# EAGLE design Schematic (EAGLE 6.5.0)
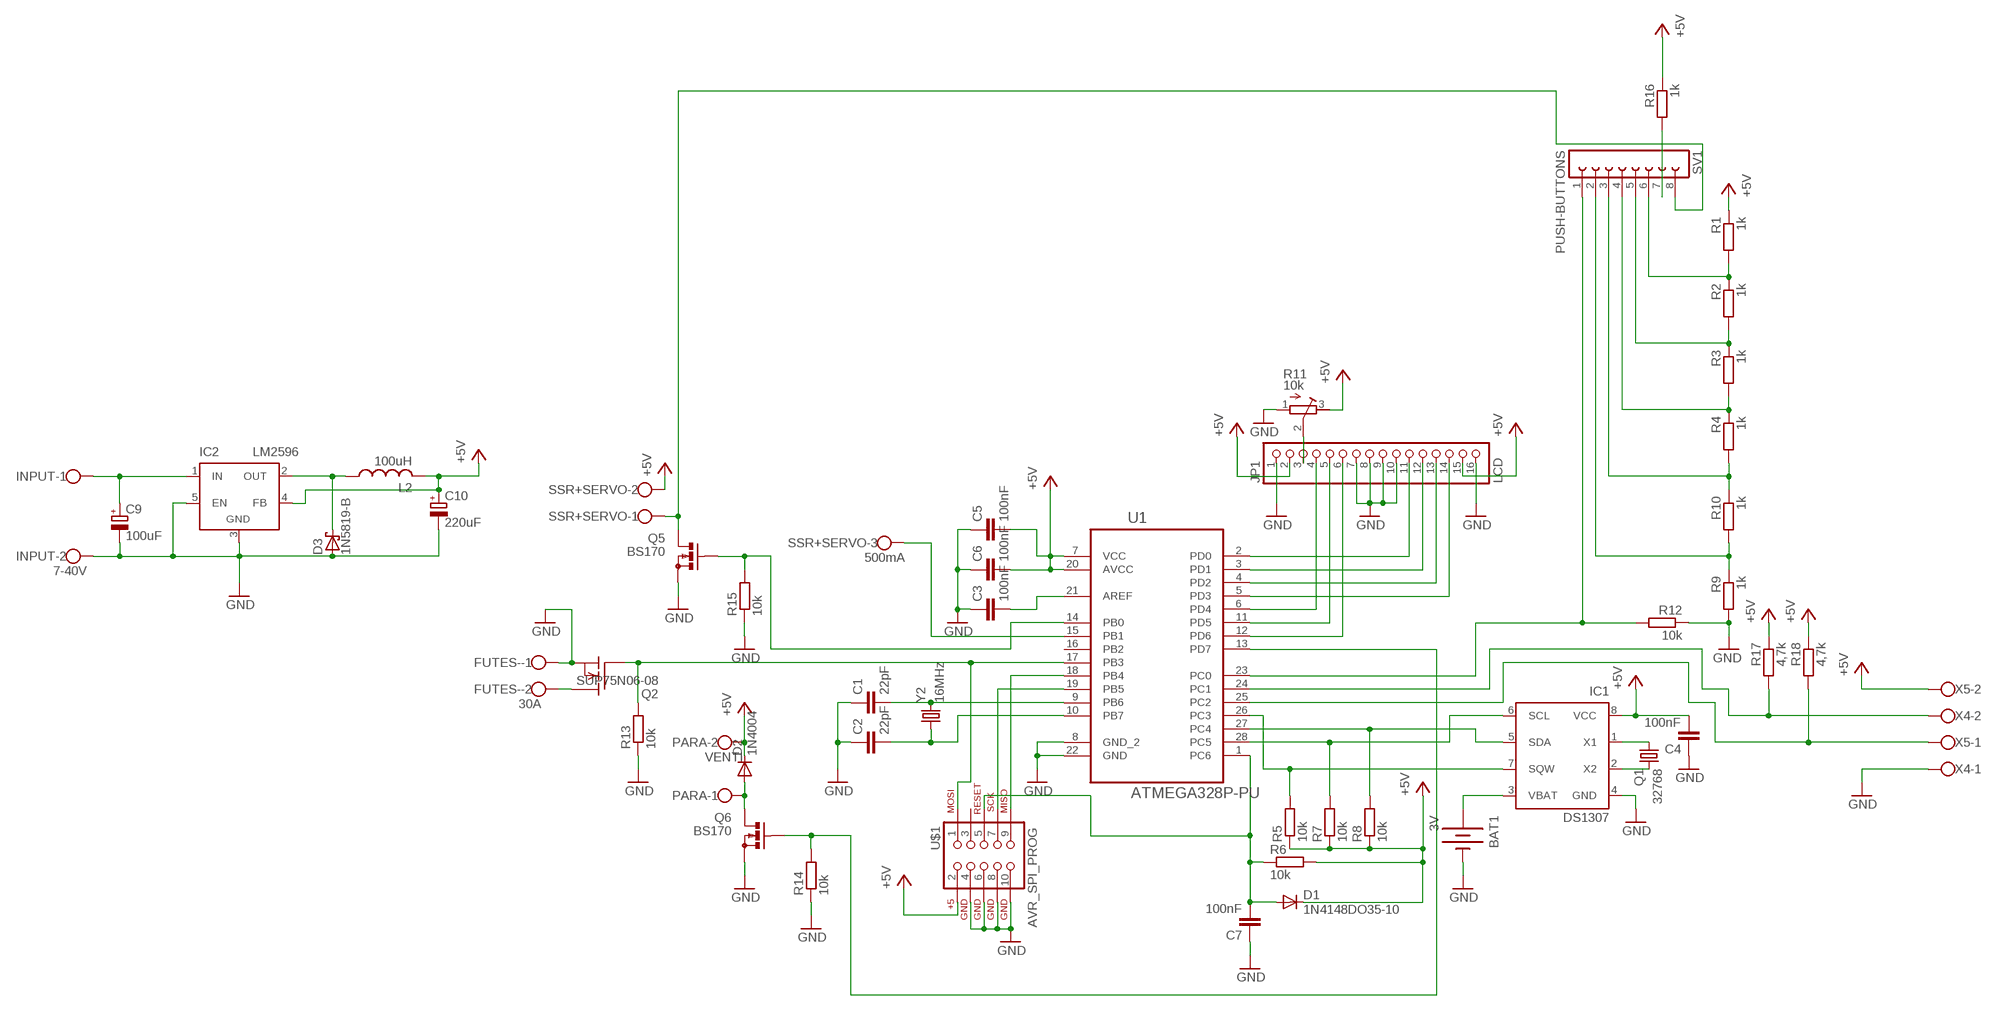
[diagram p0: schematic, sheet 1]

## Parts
BAT1  3V  BATTERY20PTH  [BATTCOM_20MM_PTH]
C1  22pF  CAPKIT  [CAP-PTH-SMALL-KIT]
C2  22pF  CAPKIT  [CAP-PTH-SMALL-KIT]
C3  100nF  CAPKIT  [CAP-PTH-SMALL-KIT]
C4  100nF  CAPKIT  [CAP-PTH-SMALL-KIT]
C5  100nF  CAPKIT  [CAP-PTH-SMALL-KIT]
C6  100nF  CAPKIT  [CAP-PTH-SMALL-KIT]
C7  100nF  CAPKIT  [CAP-PTH-SMALL-KIT]
C9  100uF  CPOL-EUE3.5-8  [E3,5-8]
C10  220uF  CPOL-EUE3.5-8  [E3,5-8]
D1  1N4148DO35-10  [DO35-10]
D2  1N4004  [DO41-10]
D3  1N5819-B  [DO41-7.6]
FUTES-  30A  W237-102  [W237-102]
IC1  DS1307  [DIL08]
IC2  LM2596  LM2596TH  [TO220-52]
INPUT  7-40V  W237-102  [W237-102]
JP1  LCD  PINHD-1X16  [1X16]
L2  100uH  L-US6000-XXX-RC  [6000-XXXX-RC]
PARA  VENTI  W237-102  [W237-102]
Q1  32768  CRYSTALTC26V  [TC26V]
Q2  SUP75N06-08  [TO220]
Q5  BS170  [SOT54E]
Q6  BS170  [SOT54E]
R1  1k  R-EU_0309/10  [0309/10]
R2  1k  R-EU_0309/10  [0309/10]
R3  1k  R-EU_0309/10  [0309/10]
R4  1k  R-EU_0309/10  [0309/10]
R5  10k  R-EU_0309/10  [0309/10]
R6  10k  R-EU_0309/10  [0309/10]
R7  10k  R-EU_0309/10  [0309/10]
R8  10k  R-EU_0309/10  [0309/10]
R9  1k  R-EU_0309/10  [0309/10]
R10  1k  R-EU_0309/10  [0309/10]
R11  10k  R-TRIMM74W  [RTRIM74W]
R12  10k  R-EU_0309/10  [0309/10]
R13  10k  R-EU_0309/10  [0309/10]
R14  10k  R-EU_0309/10  [0309/10]
R15  10k  R-EU_0309/10  [0309/10]
R16  1k  R-EU_0309/10  [0309/10]
R17  4,7k  R-EU_0309/10  [0309/10]
R18  4,7k  R-EU_0309/10  [0309/10]
SSR+SERVO  500mA  W237-103  [W237-103]
SV1  PUSH-BUTTONS  FE08-1  [FE08]
U1  ATMEGA328P-PU  [DIP254P762X457-28]
U$1  AVR_SPI_PROG  [AVR_ICSP]
X4  W237-102  [W237-102]
X5  W237-102  [W237-102]
Y2  16MHz  CRYSTALHC49US  [HC49US]

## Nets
GND: BAT1.2(-) C1.1 C2.1 C3.1 C4.1 C5.1 C6.1 C7.1 C9.- C10.- D3.A FUTES-.1 IC1.4(GND) IC2.3(GND) IC2.5(EN) INPUT.2 JP1.1 JP1.7 JP1.8 JP1.9 JP1.10 JP1.16 Q2.3(S) Q5.S Q6.S R9.2 R11.1(E) R12.1 R13.1 R14.1 R15.1 U1.8(GND_2) U1.22(GND) U$1.4 U$1.6 U$1.8 U$1.10 X4.1
N$1: IC1.6(SCL) R7.2 U1.28(PC5)
N$2: IC1.5(SDA) R8.2 U1.27(PC4)
N$3: IC1.7(SQW) R5.2 U1.26(PC3)
N$4: IC1.2(X2) Q1.2
N$5: IC1.1(X1) Q1.1
N$6: BAT1.1(+) IC1.3(VBAT)
N$7: C1.2 U1.9(PB6) Y2.2
N$8: C2.2 U1.10(PB7) Y2.1
N$9: C3.2 U1.21(AREF)
N$10: JP1.11 U1.2(PD0)
N$11: JP1.12 U1.3(PD1)
N$12: JP1.13 U1.4(PD2)
N$13: JP1.14 U1.5(PD3)
N$14: JP1.4 U1.6(PD4)
N$15: JP1.5 U1.11(PD5)
N$16: JP1.6 U1.12(PD6)
N$17: U1.18(PB4) U$1.9
N$18: C7.2 D1.A R6.1 U1.1(PC6) U$1.5
N$19: U1.19(PB5) U$1.7
N$20: Q2.1(G) R13.2 U1.17(PB3) U$1.1
N$21: C9.+ IC2.1(IN) INPUT.1
N$22: FUTES-.2 Q2.2(D)
N$23: R12.2 SV1.1 U1.23(PC0)
N$24: JP1.3 R11.2(S)
N$25: R3.2 R4.1 SV1.4
N$26: R2.2 R3.1 SV1.5
N$27: R1.2 R2.1 SV1.6
N$28: R9.1 R10.2 SV1.2
N$29: R4.2 R10.1 SV1.3
N$30: Q5.G R15.2 U1.14(PB0)
N$31: Q5.D SSR+SERVO.1 SV1.8
N$32: R16.2 SV1.7
N$33: R17.2 U1.24(PC1) X4.2
N$34: D2.A PARA.1 Q6.D
N$35: R18.2 U1.25(PC2) X5.1
N$36: SSR+SERVO.3 U1.15(PB1)
N$37: D3.C IC2.2(OUT) L2.1
N$38: Q6.G R14.2 U1.13(PD7)
VCC: C4.2 C5.2 C6.2 C10.+ D1.C D2.C IC1.8(VCC) IC2.4(FB) JP1.2 JP1.15 L2.2 PARA.2 R1.1 R5.1 R6.2 R7.1 R8.1 R11.3(A) R16.1 R17.1 R18.1 SSR+SERVO.2 U1.7(VCC) U1.20(AVCC) U$1.2 X5.2 ; supply symbol labelled +5V
Unconnected: U1.16(PB2) U$1.3

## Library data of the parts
BAT1 = SparkFun-Electromechanical:BATTERY: Battery Holders
C1-C7 = SparkFun-Capacitors:CAP: Capacitor
C9 C10 = rcl:CPOL-EU: POLARIZED CAPACITOR, European symbol
D1 = diode:1N4148: DIODE
D2 = diode:1N4004: DIODE
D3 = diode:1N581*: 1.0A SCHOTTKY BARRIER RECTIFIER
FUTES- INPUT PARA X4 X5 = con-wago-500:W237-102: WAGO SCREW CLAMP; MPN: 237-102; OC_FARNELL: unknown; OC_NEWARK: 70K9898
IC1 = ds1307_pcf8583:DS1307: I2C-Bus CLOCK/CALENDAR
IC2 = linear:LM2596T: STEP-DOWN VOLTAGE REGULATOR
JP1 = pinhead:PINHD-1X16: PIN HEADER
L2 = rcl:L-US: INDUCTOR, American symbol
Q1 = crystal:CRYSTAL: CRYSTAL; OC_FARNELL: unknown; OC_NEWARK: unknown
Q2 = transistor-fet:SUP75N06-08: N-Channel Enhancement MOSFET 60V; 75A; 0,008Ohm
Q5 Q6 = transistor-small-signal:BS170: N-CHANNEL MOS FET
R1-R10 R12-R18 = rcl:R-EU_: RESISTOR, European symbol
R11 = resistor:R-TRIMM: Trimm resistor
SSR+SERVO = con-wago-500:W237-103: WAGO SCREW CLAMP; MPN: 237-103; OC_FARNELL: unknown; OC_NEWARK: 18M7116
SV1 = con-lsta:FE08-1: FEMALE HEADER; OC_FARNELL: unknown; OC_NEWARK: unknown
U1 = Atmel_By_element14_Batch_1-00:ATMEGA328P-PU: 8-bit Microcontroller with In-System Programmable Flash; MPN: ATMEGA328P-PU; OC_FARNELL: 1715487; OC_NEWARK: 15R0268; PACKAGE: PDIP-28; SUPPLIER: Atmel
U$1 = SparkFun-Connectors:AVR_SPI_PROG: AVR 10-pin ICSP Header This is the standard AVR In Circuit Serial Programming header. Minimal, but includes pin one indicator. Works with standard Olimex programmers. Also look for the 6-pin reduced version. Spark Fun Electronics SKU: PRT-00778
Y2 = SparkFun-FreqCtrl:CRYSTAL: Various standard crystals. Proven footprints. Spark Fun Electronics SKU : COM-00534

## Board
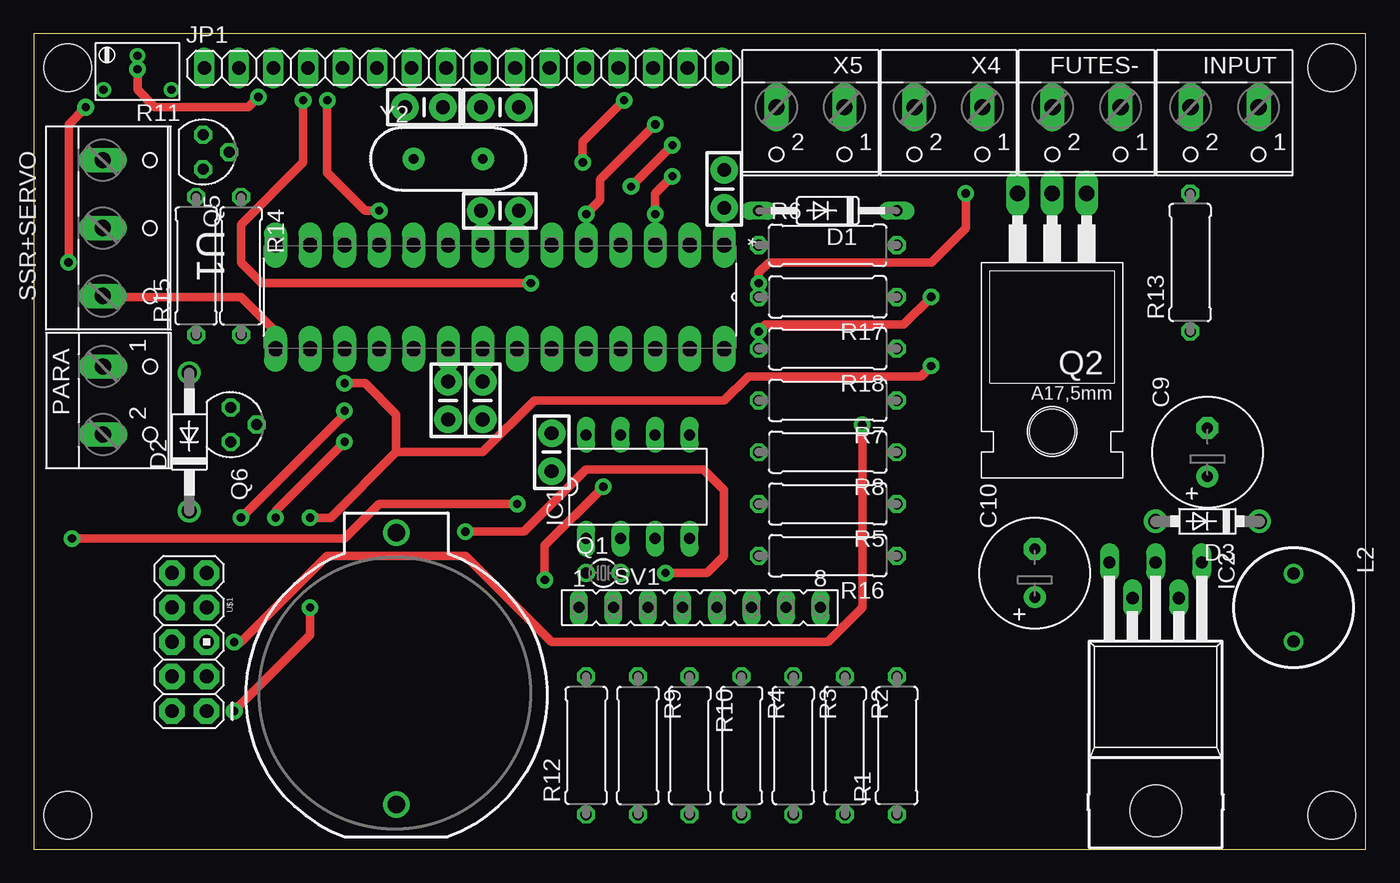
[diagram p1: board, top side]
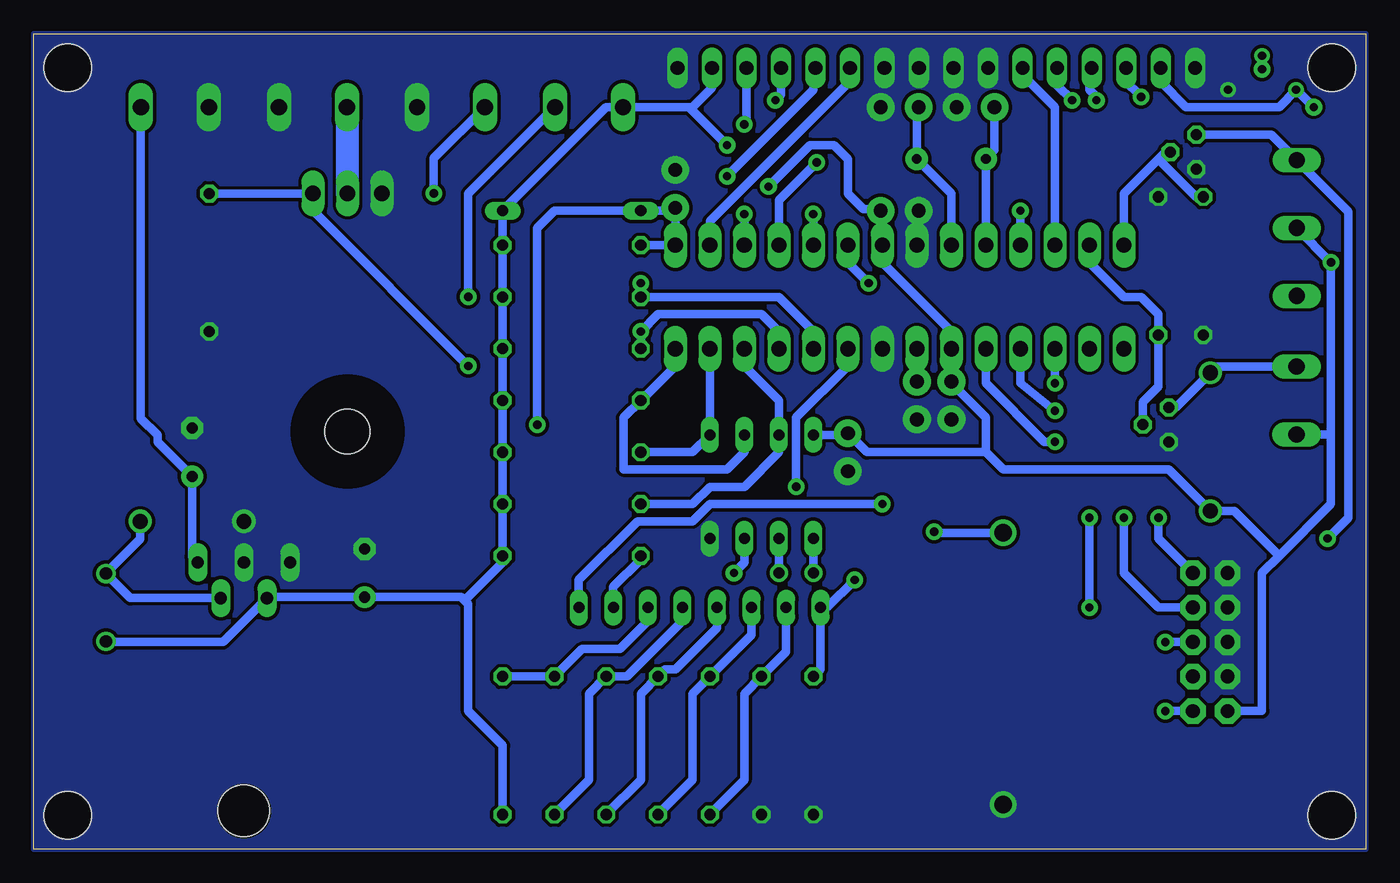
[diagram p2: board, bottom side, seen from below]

Size 98 x 60 mm. Coordinates in mm from the lower left corner, seen from the top.
Outline: 0,0 98,0 98,60 0,60 0,0
Copper layers (1*16): Top 0.035mm / dielectric 1.5mm / Bottom 0.035mm
Design rules "default *": minimum track width 24mil, minimum drill 24mil, track to track 10mil, track to pad 10mil, pad to pad 8mil, via to via 8mil, smd to smd 8mil, copper to edge 0mil, drill to drill 8mil, minimum pad ring 10mil, minimum via ring 12mil, stop-mask expansion 0mil, vias tented up to drill 0mil, thermal gap 10mil
Holes 3.5 mm at 2.5,57.5 95.5,57.5 2.5,2.5 95.5,2.5

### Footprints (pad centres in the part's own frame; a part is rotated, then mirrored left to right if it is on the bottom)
BATTCOM_20MM_PTH = drill 1.3: 1 11.85,0; 2 -8.15,0
CAP-PTH-SMALL-KIT = drill 1.016 pad 2.032: 1 -1.397,0; 2 1.397,0
E3,5-8 = drill 0.813 pad 1.6: + -1.778,0 | drill 0.813 pad 1.6 octagon: - 1.778,0
DO35-10 = drill 0.813 long: A 5.08,0; C -5.08,0
DO41-10 = drill 1.118: A 5.08,0; C -5.08,0
DO41-7.6 = drill 1.1 pad 1.7: A 3.81,0; C -3.81,0
W237-102 = drill 1.194 long: 1 -2.5,-1.27; 2 2.5,-1.27
DIL08 = drill 0.813 long: 1 -3.81,-3.81; 2 -1.27,-3.81; 3 1.27,-3.81; 4 3.81,-3.81; 5 3.81,3.81; 6 1.27,3.81; 7 -1.27,3.81; 8 -3.81,3.81
TO220-52 = drill 0.9 long: 1 -3.4,-21.1; 2 -1.7,-18.47; 3 0,-21.1; 4 1.7,-18.47; 5 3.4,-21.1 | hole 3.8: 0,-2.8
1X16 = drill 1.016 long: 1 -19.05,0; 2 -16.51,0; 3 -13.97,0; 4 -11.43,0; 5 -8.89,0; 6 -6.35,0; 7 -3.81,0; 8 -1.27,0; 9 1.27,0; 10 3.81,0; 11 6.35,0; 12 8.89,0; 13 11.43,0; 14 13.97,0; 15 16.51,0; 16 19.05,0
6000-XXXX-RC = drill 0.9 pad 1.422: 1 -2.5,0; 2 2.5,0
TC26V = drill 0.813: 1 -1.27,0; 2 1.27,0
TO220 = drill 1.118 long: 1 -2.54,-6.35; 2 0,-6.35; 3 2.54,-6.35 | hole 3.302: 0,11.176
SOT54E = drill 0.813 octagon: D -1.27,0; G 0,1.905; S 1.27,0
0309/10 = drill 0.813 octagon: 1 -5.08,0; 2 5.08,0
RTRIM74W = drill 0.61: 1 -1.25,-2.5; 2 1.25,0; 3 -1.25,2.5
W237-103 = drill 1.194 long: 1 -5,-1.29; 2 0,-1.29; 3 5,-1.29
FE08 = drill 0.813 long: 1 -8.89,0; 2 -6.35,0; 3 -3.81,0; 4 -1.27,0; 5 1.27,0; 6 3.81,0; 7 6.35,0; 8 8.89,0
DIP254P762X457-28 = drill 1.118 long: 1 -7.62,33.02; 2 -7.62,30.48; 3 -7.62,27.94; 4 -7.62,25.4; 5 -7.62,22.86; 6 -7.62,20.32; 7 -7.62,17.78; 8 -7.62,15.24; 9 -7.62,12.7; 10 -7.62,10.16; 11 -7.62,7.62; 12 -7.62,5.08; 13 -7.62,2.54; 14 -7.62,0; 15 0,0; 16 0,2.54; 17 0,5.08; 18 0,7.62; 19 0,10.16; 20 0,12.7; 21 0,15.24; 22 0,17.78; 23 0,20.32; 24 0,22.86; 25 0,25.4; 26 0,27.94; 27 0,30.48; 28 0,33.02
AVR_ICSP = drill 1.016 pad 1.88 octagon: 1 -1.27,5.08; 2 1.27,5.08; 3 -1.27,2.54; 4 1.27,2.54; 5 -1.27,0; 6 1.27,0; 7 -1.27,-2.54; 8 1.27,-2.54; 9 -1.27,-5.08; 10 1.27,-5.08
HC49US = drill 0.7 pad 1.651: 1 -2.54,0; 2 2.54,0

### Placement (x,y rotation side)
BAT1  26.67,11.43 90 top
C1  34.29,54.61 180 top
C2  28.7,54.61 180 top
C3  33.02,33.02 90 top
C4  38.1,29.21 90 top
C5  34.29,46.99 0 top
C6  30.48,33.02 90 top
C7  50.8,48.59 270 top
C9  86.36,29.21 90 top
C10  73.66,20.32 90 top
D1  58.42,46.99 180 top
D2  11.43,29.97 90 top
D3  86.36,24.13 180 top
FUTES-  77.47,53.34 180 top
IC1  44.45,26.67 0 top
IC2  82.55,0 180 top
INPUT  87.63,53.34 180 top
JP1  31.59,57.5 0 top
L2  92.71,17.78 270 top
PARA  6.35,33.02 270 top
Q1  41.91,20.32 0 top
Q2  74.93,41.91 180 top
Q5  12.45,51.31 270 top
Q6  14.48,31.24 270 top
R1  63.5,7.62 90 top
R2  59.69,7.62 270 top
R3  55.88,7.62 270 top
R4  52.07,7.62 270 top
R5  58.42,25.4 180 top
R6  58.42,44.45 0 top
R7  58.42,33.02 180 top
R8  58.42,29.21 180 top
R9  44.45,7.62 270 top
R10  48.26,7.62 270 top
R11  7.62,57.15 90 top
R12  40.64,7.62 90 top
R13  85.09,43.18 90 top
R14  15.24,42.93 270 top
R15  11.94,42.93 90 top
R16  58.42,21.59 180 top
R17  58.42,40.64 180 top
R18  58.42,36.83 180 top
SSR+SERVO  6.35,45.72 270 top
SV1  49,17.78 0 top
U1  17.78,36.83 270 top
U$1  11.43,15.24 180 top
X4  67.31,53.34 180 top
X5  57.15,53.34 180 top
Y2  30.48,50.8 0 top

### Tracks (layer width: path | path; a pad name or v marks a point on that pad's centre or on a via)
GND
  pour Bottom (no thermals): 0,0 0,60 98,60 98,0
N$1
  Bottom 0.61: IC1.6 45.72,29.21 46.99,27.94 54.61,27.94 54.61,31.75 R7.2 50.8,35.56 U1.28
N$2
  Bottom 0.61: U1.27 IC1.5 49.53,29.21 R8.2
N$3
  Bottom 0.61: U1.26 45.72,35.56 43.18,33.02 IC1.7 43.18,29.21 45.72,26.67 48.26,26.67 49.53,25.4 R5.2
N$4
  Bottom 0.61: IC1.2 Q1.2
N$5
  Bottom 0.61: IC1.1 Q1.1
N$6  (via drill 0.61)
  Top 0.61: v46.48,20.32 49.53,20.32 50.8,21.59 50.8,26.42 49.28,27.94 40.64,27.94 36.07,23.37 v31.75,23.37
  Bottom 0.61: IC1.3 45.72,21.08 v46.48,20.32 | BAT1.1 31.66,23.28 v31.75,23.37
N$7
  Bottom 0.61: C1.2 33.02,54.61 Y2.2 30.48,48.26 U1.9
N$8
  Bottom 0.61: 28.07,50.93 Y2.1 | Y2.1 U1.10 | C2.2 27.3,51.44 Y2.1
N$9
  Bottom 0.61: U1.21 C3.2 33.02,34.29
N$10
  Bottom 0.61: U1.2 48.26,46.23 38.1,56.39 38.1,57.34 JP1.11 38.1,57.15
N$11  (via drill 0.61)
  Top 0.61: v45.72,46.74 45.72,48.26 v46.99,49.53
  Bottom 0.61: JP1.12 40.64,57.15 40.64,55.88 v46.99,49.53 | U1.3 v45.72,46.74
N$12  (via drill 0.61)
  Top 0.61: v40.39,50.55 40.39,52.07 v43.43,55.12
  Bottom 0.61: v40.39,50.55 43.18,47.75 U1.4 | JP1.13 43.02,55.53 v43.43,55.12
N$13  (via drill 0.61)
  Top 0.61: v45.72,53.34 41.66,49.28 41.66,47.75 v40.64,46.74
  Bottom 0.61: JP1.14 45.56,53.5 v45.72,53.34 | v40.64,46.74 U1.5
N$14  (via drill 0.61)
  Top 0.61: v36.58,41.66 16.76,41.66 15.24,43.18 15.24,45.97 19.81,50.55 v19.81,55.12
  Bottom 0.61: U1.6 38.1,43.18 v36.58,41.66 | v19.81,55.12 19.81,55.37 20.32,55.88 20.32,57.34 JP1.4
N$15  (via drill 0.61)
  Top 0.61: v25.4,46.99 24.38,46.99 21.59,49.78 v21.59,55.12
  Bottom 0.61: v25.4,46.99 U1.11 | JP1.5 22.7,56.23 v21.59,55.12
N$16
  Bottom 0.61: JP1.6 25.4,57.15 22.86,54.61 U1.12
N$17  (via drill 0.61)
  Top 0.61: v22.86,32.26 22.86,32 v15.24,24.38
  Bottom 0.61: U1.18 25.4,34.29 v22.86,32.26 | v15.24,24.38 15.24,22.86 U$1.9
N$18  (via drill 0.61)
  Top 0.61: v60.96,31.24 60.96,17.78 58.42,15.24 38.1,15.24 31.75,21.59 21.59,21.59 15.24,15.24 v14.73,15.24
  Bottom 0.61: U$1.5 v14.73,15.24 | v60.96,31.24 60.96,45.72 59.69,46.99 D1.A 51.01,46.99 C7.2 U1.1 R6.1
N$19  (via drill 0.61)
  Top 0.61: v17.78,24.38 17.78,24.89 v22.86,29.97
  Bottom 0.61: v17.78,24.38 17.78,20.32 15.24,17.78 U$1.7 | v22.86,29.97 23.62,29.97 27.94,34.29 U1.19
N$20  (via drill 0.61)
  Top 0.61: 26.67,29.21 33.02,29.21 36.83,33.02 50.8,33.02 52.58,34.8 65.28,34.8 v66.04,35.56 | v20.32,17.78 20.32,15.75 v14.73,10.16 | v20.32,24.38 21.84,24.38 26.67,29.21 | 26.67,29.21 26.67,32 24.38,34.29 v22.86,34.29
  Bottom 0.61: v20.32,24.38 v20.32,17.78 | v14.73,10.16 U$1.1 | R13.2 Q2.1 77.47,46.99 v66.04,35.56 | v22.86,34.29 U1.17
N$21
  Bottom 0.61: IC2.1 86.36,21.51 C9.+ 88.9,29.97 88.9,30.48 90.13,31.71 INPUT.1
N$22
  Bottom 0.61: 74.93,54.61 FUTES-.2
  Bottom 1.676: Q2.2 74.93,54.57 FUTES-.2
N$23  (via drill 0.61)
  Top 0.61: v37.59,19.81 37.59,22.35 v41.91,26.67
  Bottom 0.61: U1.23 38.1,35.56 41.91,31.75 v41.91,26.67 | R12.2 40.11,13.23 SV1.1 39.62,17.78 v37.59,19.81
N$24  (via drill 0.61)
  Top 0.61: v7.62,57.4 7.62,55.88 8.89,54.61 15.75,54.61 v16.51,55.37
  Bottom 0.61: R11.2 v7.62,57.4 | v16.51,55.37 17.78,56.64 17.78,57.34 JP1.3
N$25
  Bottom 0.61: R3.2 53.34,5.08 53.34,11.43 R4.1 51.56,13.21 50.8,13.21 47.73,16.28 SV1.4
N$26
  Bottom 0.61: R2.2 57.15,5.08 57.15,11.43 R3.1 54.36,12.7 50.27,16.79 SV1.5
N$27
  Bottom 0.61: R1.2 R2.1 57.66,14.73 54.86,14.73 52.81,16.79 SV1.6
N$28
  Bottom 0.61: SV1.2 42.65,14.5 R9.1 45.72,11.43 45.72,5.08 R10.2
N$29
  Bottom 0.61: SV1.3 45.19,15.77 R10.1 49.53,11.43 49.53,5.08 R4.2
N$30
  Bottom 0.61: Q5.G 14.73,51.31 15.24,50.8 | 15.24,50.8 17.78,48.26 U1.14 | R15.2 12.45,48.01 15.24,50.8
N$31  (via drill 0.61)
  Top 0.61: v35.56,25.4 25.4,25.4 22.86,22.86 v2.79,22.86
  Bottom 0.61: v35.56,25.4 48.26,25.4 49.53,24.13 53.59,24.13 57.91,19.81 57.91,17.8 SV1.8 | 5.08,50.7 SSR+SERVO.1 | Q5.D 6.92,52.58 SSR+SERVO.1 | SSR+SERVO.1 1.27,46.93 1.27,24.38 v2.79,22.86
N$32
  Bottom 0.61: R16.2 53.34,21.34 55.37,19.3 55.37,17.8 SV1.7
N$33  (via drill 0.61)
  Top 0.61: v68.58,48.26 68.58,45.72 66.04,43.18 54.1,43.18 53.34,42.42 v53.34,41.66
  Bottom 0.61: U1.24 40.64,38.1 43.18,40.64 R17.2 v53.34,41.66 | v68.58,48.26 68.58,50.84 X4.2
N$34
  Bottom 0.61: PARA.1 10.96,35.52 D2.A 13.97,32.51 Q6.D
N$35  (via drill 0.61)
  Top 0.61: v66.04,40.64 64.01,38.61 53.85,38.61 v53.34,38.1
  Bottom 0.61: R18.2 v53.34,38.1 52.07,39.37 44.45,39.37 43.18,38.1 U1.25 | X5.1 59.69,54.61 66.04,48.26 v66.04,40.64
N$36
  Top 0.61: 5.08,40.64 SSR+SERVO.3 5.14,40.64 15.24,40.64 17.78,38.1 U1.15
N$37
  Bottom 0.61: IC2.2 90.9,18.47 L2.1 90.17,22.82 D3.C
N$38
  Bottom 0.61: U1.13 20.32,43.18 17.78,40.64 16.51,40.64 15.24,39.37 R14.2 15.24,34.04 16.38,32.89 Q6.G
VCC  (via drill 0.61)
  Top 0.61: v43.94,48.77 v46.99,51.82 | v2.54,43.18 2.54,53.34 v3.81,54.61
  Bottom 0.61: IC1.8 38.1,30.48 C4.2 36.7,29.21 27.94,29.21 | 35.56,43.18 30.48,38.1 U1.20 C6.2 30.48,34.29 27.94,31.75 27.94,29.21 | U1.7 35.56,43.18 | 5.08,55.88 6.35,54.61 13.21,54.61 15.08,56.48 JP1.2 | v3.81,54.61 5.08,55.88 | 5.08,55.88 R11.3 | 49.78,54.61 X5.2 55.88,54.61 D1.C 63.5,45.72 R6.2 R17.1 R18.1 R7.1 R8.1 R5.1 R16.1 63.5,21.08 66.29,18.29 | 49.78,54.61 49.53,54.61 48.1,56.04 JP1.15 | L2.2 92.71,15.24 84.08,15.24 81.41,17.91 | U$1.2 7.62,10.16 7.62,20.32 6.35,21.59 | 81.41,17.91 IC2.4 | R1.1 63.5,7.62 66.04,10.16 66.04,18.03 66.29,18.29 | 66.29,18.29 66.55,18.54 C10.+ 80.52,18.54 81.28,17.78 81.41,17.91 | 35.56,43.18 35.69,43.31 C5.2 35.69,47.12 36.96,47.12 38.1,48.26 38.1,50.8 39.12,51.82 40.89,51.82 v43.94,48.77 | v46.99,51.82 49.78,54.61 | 6.35,21.59 2.54,25.4 2.54,30.48 | PARA.2 2.58,30.52 2.54,30.48 | 27.94,29.21 26.67,27.94 14.48,27.94 D2.C 9.65,24.89 6.35,21.59 | 2.54,30.48 v2.54,43.18 5.06,45.7 SSR+SERVO.2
